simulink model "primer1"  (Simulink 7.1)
settings: Solver=FixedStepDiscrete  StartTime=0.0  StopTime=5e-6  RelTol=1e-3
undefined symbols (not defined in the file or in its folder): interp1
libraries: powerlib x18

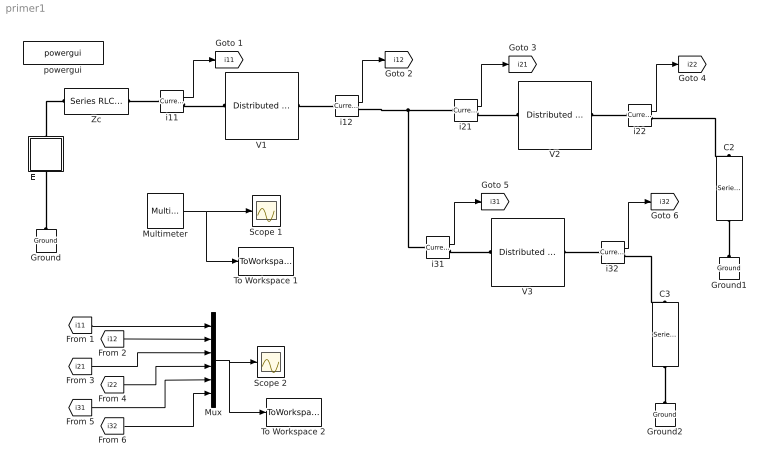
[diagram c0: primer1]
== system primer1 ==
  C2 : powerlib/Elements/Series RLC Branch  Orientation=down  DialogController=POWERSYS.PowerSysDialog  PhysicalDomain=powersysdomain  SubClassName=unknown  LeftPortType=p1  RightPortType=p1  LConnTagsString=__new0  RConnTagsString=__new0  BranchType=C  Resistance=400  Inductance=1e-3  SetiL0=off  InitialCurrent=0  Capacitance=2e-9  Setx0=on  InitialVoltage=0  Measurements=None
  C3 : powerlib/Elements/Series RLC Branch  Orientation=down  DialogController=POWERSYS.PowerSysDialog  PhysicalDomain=powersysdomain  SubClassName=unknown  LeftPortType=p1  RightPortType=p1  LConnTagsString=__new0  RConnTagsString=__new0  BranchType=C  Resistance=400  Inductance=1e-3  SetiL0=off  InitialCurrent=0  Capacitance=2e-9  Setx0=on  InitialVoltage=0  Measurements=None
  E : Subsystem  Orientation=up  mask(Proizvolen generator){vreme=[0 0.001 0.5 0.501 50]/1e6, napon=2*[0 500 500 0 0]*1000}
      mask prompts: vreme "Vreme (s)"; napon "Napon (V)"
      mask help: So ovoj element e definiran idealen naponski generator so proizvolen oblik. Oblikot na naponot se definira so pomos na dva vektori, pri sto vo prviot vektor se dadeni diskretni vremenski momenti dodeka vrednostite na naponot vo tie momenti se dadeni vo vtoriot vektor. Za ostanatite vremenski momenti koi sto ne se dadeni vo vektorite modelot pravi linearna interpolacija.
  Ground : powerlib/Elements/Ground  Orientation=down  DialogController=POWERSYS.PowerSysDialog  PhysicalDomain=powersysdomain  SubClassName=unknown  LeftPortType=p1  RightPortType=p1  LConnTagsString=a
  Ground1 : powerlib/Elements/Ground  Orientation=down  DialogController=POWERSYS.PowerSysDialog  PhysicalDomain=powersysdomain  SubClassName=unknown  LeftPortType=p1  RightPortType=p1  LConnTagsString=a
  Ground2 : powerlib/Elements/Ground  Orientation=down  DialogController=POWERSYS.PowerSysDialog  PhysicalDomain=powersysdomain  SubClassName=unknown  LeftPortType=p1  RightPortType=p1  LConnTagsString=a
  Multimeter : powerlib/Measurements/Multimeter  SystemSampleTime=-1  PhasorSimulation=off  OutputType=Complex  sel=[1 2 3 4 5 6]  L=7  Gain=[1 1 1 1 1 1]  yselected={'Us_ph1_gnd: V1','Ur_ph1_gnd: V1','Us_ph1_gnd: V2','Ur_ph1_gnd: V2','Us_ph1_gnd: V3','Ur_ph1_gnd: V3'};  PSBOutputType=1  PSBequivalent=0  AxesSetting=[0,0.1,-100,100]  Display=0  SavedBlockNames=-11
  Mux : Mux  Inputs=6
  Scope 1 : Scope
  Scope 2 : Scope
  To Workspace 1 : ToWorkspace  VariableName=naponi  SampleTime=-1  SaveFormat=Structure With Time
  To Workspace 2 : ToWorkspace  VariableName=strui  SampleTime=-1  SaveFormat=Structure With Time
  V1 : powerlib/Elements/Distributed Parameters Line  DialogController=POWERSYS.PowerSysDialog  SystemSampleTime=-1  Phases=1  Frequency=50  Resistance=0.001  Inductance=1.334e-3  Capacitance=8.334e-009  Length=0.3  x1=[0 0;2.00057995591278e-007 0;4.00115991182557e-007 0;6.00173986773835e-007 0;8.00231982365114e-007 0;1.00028997795639e-006 0]  x2=[0 0;2.00057995591278e-007 0;4.00115991182557e-007 0;6.00173986773835e-007 0;8.00231982365114e-007 0;1.00028997795639e-006 0]  x3=[0 0;2.00057995591278e-007 0;4.00115991182557e-007 0;6.00173986773835e-007 0;8.00231982365114e-007 0;1.00028997795639e-006 0]  x4=[0 0;2.00057995591278e-007 0;4.00115991182557e-007 0;6.00173986773835e-007 0;8.00231982365114e-007 0;1.00028997795639e-006 0]  x5=1.00028997795639e-006  Measurements=Phase-to-ground voltages
  V2 : powerlib/Elements/Distributed Parameters Line  DialogController=POWERSYS.PowerSysDialog  SystemSampleTime=-1  Phases=1  Frequency=50  Resistance=0.001  Inductance=1.334e-3  Capacitance=8.334e-009  Length=0.03  x1=[0 0;2.00057995591278e-008 0;4.00115991182557e-008 0;6.00173986773835e-008 0;8.00231982365114e-008 0;1.00028997795639e-007 0]  x2=[0 0;2.00057995591278e-008 0;4.00115991182557e-008 0;6.00173986773835e-008 0;8.00231982365114e-008 0;1.00028997795639e-007 0]  x3=[0 0;2.00057995591278e-008 0;4.00115991182557e-008 0;6.00173986773835e-008 0;8.00231982365114e-008 0;1.00028997795639e-007 0]  x4=[0 0;2.00057995591278e-008 0;4.00115991182557e-008 0;6.00173986773835e-008 0;8.00231982365114e-008 0;1.00028997795639e-007 0]  x5=1.00028997795639e-007  Measurements=Phase-to-ground voltages
  V3 : powerlib/Elements/Distributed Parameters Line  DialogController=POWERSYS.PowerSysDialog  SystemSampleTime=-1  Phases=1  Frequency=50  Resistance=0.001  Inductance=1.334e-3  Capacitance=8.334e-009  Length=0.06  x1=[0 0;4.00115991182557e-008 0;8.00231982365114e-008 0;1.20034797354767e-007 0;1.60046396473023e-007 0;2.00057995591278e-007 0]  x2=[0 0;4.00115991182557e-008 0;8.00231982365114e-008 0;1.20034797354767e-007 0;1.60046396473023e-007 0;2.00057995591278e-007 0]  x3=[0 0;4.00115991182557e-008 0;8.00231982365114e-008 0;1.20034797354767e-007 0;1.60046396473023e-007 0;2.00057995591278e-007 0]  x4=[0 0;4.00115991182557e-008 0;8.00231982365114e-008 0;1.20034797354767e-007 0;1.60046396473023e-007 0;2.00057995591278e-007 0]  x5=2.00057995591278e-007  Measurements=Phase-to-ground voltages
  Zc : powerlib/Elements/Series RLC Branch  DialogController=POWERSYS.PowerSysDialog  PhysicalDomain=powersysdomain  SubClassName=unknown  LeftPortType=p1  RightPortType=p1  LConnTagsString=__new0  RConnTagsString=__new0  BranchType=R  Resistance=400  Inductance=1e-3  SetiL0=off  InitialCurrent=0  Capacitance=2e-9  Setx0=on  InitialVoltage=0  Measurements=None
  i{11..12,21..22,31..32} (6 alike) : powerlib/Measurements/Current Measurement  DialogController=POWERSYS.PowerSysDialog  SystemSampleTime=-1  PhasorSimulation=off  OutputType=Complex  PSBequivalent=0
  powergui : powerlib/powergui  SystemSampleTime=-1  SimulationMode=Discrete  SampleTime=10e-9  frequency=60  SPID=off  SwTol=0  Interpol=off  x0status=blocks  echomessages=off  HookPort=off  FunctionMessages=off  EnableUseOfTLC=off  RestoreLinks=warning  frequencyindice=0  Frange=[0:2:500]  Ylog=off  Xlog=on  ShowGrid=off  save=off  variable=ZData  ZoomFFT=on  StartTime=0.0  cycles=1  DisplayStyle=1  fundamental=60  FreqAxis=off  MaxFrequency=1000  frequencyindicesteady=1  RmsSteady=1  display=off  Ts=0  methode=off
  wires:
  Multimeter/1 -> Scope 1/1, To Workspace 1/1
  i11/1 -> [i11]
  i12/1 -> [i12]
  i22/1 -> [i22]
  i21/1 -> [i21]
  i32/1 -> [i32]
  i31/1 -> [i31]
  Mux/1 -> Scope 2/1, To Workspace 2/1
  [i11] -> Mux/1
  [i12] -> Mux/2
  [i21] -> Mux/3
  [i22] -> Mux/4
  [i31] -> Mux/5
  [i32] -> Mux/6
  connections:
  Ground/LConn1 -- E/LConn1
  E/RConn1 -- Zc/LConn1
  C2/RConn1 -- Ground1/LConn1
  Zc/RConn1 -- i11/LConn1
  i11/RConn1 -- V1/LConn1
  V1/RConn1 -- i12/LConn1
  i31/LConn1 -- i12/RConn1 -- i21/LConn1
  i21/RConn1 -- V2/LConn1
  V2/RConn1 -- i22/LConn1
  i31/RConn1 -- V3/LConn1
  V3/RConn1 -- i32/LConn1
  C3/RConn1 -- Ground2/LConn1
  i22/RConn1 -- C2/LConn1
  i32/RConn1 -- C3/LConn1

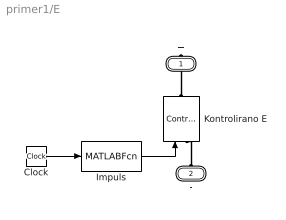
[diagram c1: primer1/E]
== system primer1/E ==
  Clock : Clock
  Impuls : MATLABFcn  MATLABFcn=interp1(vreme, napon, u)  OutputSignalType=real
  Kontrolirano E : powerlib/Electrical Sources/Controlled Voltage Source  Orientation=up  DialogController=POWERSYS.PowerSysDialog  SystemSampleTime=-1  Initialize=on  Source_Type=AC  Amplitude=0  Phase=0  Frequency=0  Measurements=Voltage
  + : PMIOPort  Orientation=down  Port=1  Side=Right
  - : PMIOPort  Orientation=up  Port=2  Side=Left
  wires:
  Impuls/1 -> Kontrolirano E/1
  Clock/1 -> Impuls/1
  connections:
  +/RConn1 -- Kontrolirano E/RConn1
  -/RConn1 -- Kontrolirano E/LConn1
